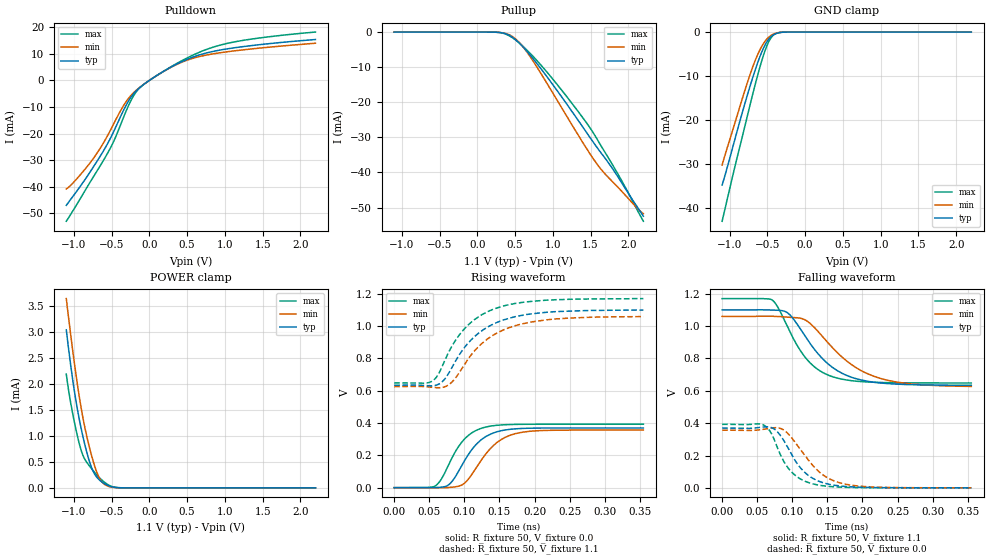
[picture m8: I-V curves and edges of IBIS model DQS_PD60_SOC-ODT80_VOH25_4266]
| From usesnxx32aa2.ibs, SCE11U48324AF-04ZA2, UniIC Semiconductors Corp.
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| DQS_PD60_SOC-ODT80_VOH25_4266
| (60 Ohm Pulldown, 80 Ohm System ODT Setting, VOH=VDDQ/2.5, 3200-4266Mbps)
[Model]   DQS_PD60_SOC-ODT80_VOH25_4266
Model_type   I/O
Vinl = 160.000mV
Vinh = 280.000mV
Vmeas = 220.000mV
Vref = 0.0mV
Cref = 0.0pF
Rref = 80.000Ohm
|   typ   min   max
|C_comp   0.838pF   0.788pF   0.888pF
C_comp_pullup   0.4190pF   0.3940pF   0.4440pF
C_comp_pulldown   0.4190pF   0.3940pF   0.4440pF
| Note: C_comp changes when the ODT circuit is enabled.
[Model Spec]
| Input threshold voltage corners
Vinl   0.1600V   0.1520V   0.1740V
Vinh   0.2800V   0.2720V   0.2940V
| Measurement voltage corners
Vmeas   0.2200V   0.2120V   0.2340V
| Timing spec test load voltage corners
Vref   0.0000V   0.0000V   0.0000V
| Dynamic Overshoot Parameters from LPDDR4 Specification
D_overshoot_ampl_h   0.30   NA   NA
D_overshoot_ampl_l   0.30   NA   NA
D_overshoot_area_h   0.1n   NA   NA
D_overshoot_area_l   0.1n   NA   NA
[Receiver Thresholds]
Vcross_low   = 160.0mV
Vcross_high  = 280.0mV
Vdiff_ac   = 120mV
Vdiff_dc   = 120mV
Tdiffslew_ac = 10.000ns |Not specified, so set to high value
[Voltage Range]   1.1000V   1.0600V   1.1700V
[Pullup Reference]   1.1000V   1.0600V   1.1700V
| Junction Temperature (Ambient temp is 35C typ 95C min -40C max)
[Temperature Range]   50.0   110.0   -40.0
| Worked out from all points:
|   slope of the pulldown table from 0 to 0.165 V, typ, clamps not added: 54.7 ohm
|   slope of the pullup table from 0 to 0.165 V, typ, clamps not added: 16.4 kohm
|   GND clamp passes 1 mA (typ) near -0.45 V on its own axis
|   POWER clamp passes 1 mA (typ) near -0.88 V on its own axis
|   rising waveform, R_fixture 50, V_fixture 0.0: 20-80 % time 35.8ps typ, 39.3ps min, 32.8ps max; typ from 0.001 V to 0.37 V
|   falling waveform, R_fixture 50, V_fixture 1.1: 20-80 % time 55.5ps typ, 67.8ps min, 44.8ps max; typ from 1.1 V to 0.634 V
|   rising waveform, R_fixture 50, V_fixture 1.1: 20-80 % time 57.8ps typ, 60.8ps min, 54.6ps max; typ from 0.634 V to 1.1 V
|   falling waveform, R_fixture 50, V_fixture 0.0: 20-80 % time 36.3ps typ, 43.3ps min, 31.1ps max; typ from 0.37 V to 0.001 V
[Pulldown]
|   Voltage   I(typ)   I(min)   I(max)
-1.1V     -46.99mA   -40.8mA    -52.96mA
-786.5mV  -34.49mA   -31.05mA   -38.36mA
-641.3mV  -28.08mA   -25.11mA   -31.66mA
-525.8mV  -22.32mA   -19.3mA    -25.97mA
-367.4mV  -12.77mA   -10.72mA   -15.73mA
-258.5mV  -6.989mA   -6.176mA   -8.45mA
-162.8mV  -3.638mA   -3.468mA   -3.924mA
-63.8mV   -1.314mA   -1.293mA   -1.298mA
414.7mV   6.826mA    6.638mA    7.153mA
847mV     10.89mA    9.975mA    12.5mA
1.375V    13.14mA    11.88mA    15.61mA
2.2V      15.36mA    13.96mA    18.16mA
[GND Clamp]
|   Voltage   I(typ)   I(min)   I(max)
-1.1V     -34.89mA   -30.34mA   -43.14mA
-935mV    -24.72mA   -20.96mA   -31.01mA
-803mV    -16.58mA   -13.55mA   -21.77mA
-733.7mV  -12.55mA   -9.876mA   -16.88mA
-667.7mV  -8.943mA   -6.74mA    -12.35mA
-591.8mV  -5.274mA   -3.797mA   -7.53mA
-519.2mV  -2.572mA   -1.835mA   -3.676mA
-463.1mV  -1.239mA   -899.6uA   -1.602mA
-410.3mV  -534.6uA   -395.8uA   -582.2uA
-341mV    -134.1uA   -102.7uA   -114.3uA
-242mV    -10.14uA   -9.274uA   -5.696uA
2.2V      0A         0A         0A
[Pullup]
|   Voltage   I(typ)   I(min)   I(max)
-1.1V     4.112uA    7.441uA    1.363uA
259.6mV   -60.64uA   -60.03uA   -61.53uA
388.3mV   -576.1uA   -480.7uA   -688.2uA
500.5mV   -2.042mA   -1.831mA   -2.144mA
609.4mV   -4.304mA   -4.305mA   -4.133mA
731.5mV   -7.378mA   -7.995mA   -6.76mA
1.045V    -16.3mA    -18.97mA   -14.58mA
1.448V    -28.62mA   -33.18mA   -25.89mA
1.573V    -32.49mA   -37.21mA   -29.99mA
1.695V    -36.01mA   -40.47mA   -34.38mA
1.91V     -42.82mA   -45.28mA   -42.24mA
2.2V      -52.46mA   -51.74mA   -53.91mA
[POWER Clamp]
|   Voltage   I(typ)   I(min)   I(max)
-1.1V     3.036mA    3.636mA    2.186mA
-1.041V   2.347mA    2.931mA    1.626mA
-981.2mV  1.754mA    2.277mA    1.183mA
-911.9mV  1.201mA    1.611mA    764.7uA
-852.5mV  818.9uA    1.149mA    543.6uA
-776.6mV  434.4uA    683.5uA    390.2uA
-710.6mV  232.2uA    359.1uA    273.1uA
-657.8mV  146.8uA    178.8uA    190.7uA
-595.1mV  80.84uA    68.31uA    109.3uA
-492.8mV  18.88uA    11.58uA    24.06uA
-380.6mV  1.613uA    1.137uA    1.355uA
2.2V      0A         0A         0A
[Ramp]
|   typ   min   max
| 20% - 80%
dV/dt_r   221.49m/35.79p   213.85m/39.28p   235.57m/32.78p
dV/dt_f   279.40m/55.49p   259.55m/67.76p   312.92m/44.82p
| 25% - 75%
|dV/dt_r   184.57m/28.53p   178.21m/31.31p   196.31m/26.01p
|dV/dt_f   232.84m/44.18p   216.29m/54.01p   260.77m/35.67p
R_load = 50
[Rising Waveform]
R_fixture = 50
V_fixture = 0.0
|   Time   V(typ)   V(min)   V(max)
0s        730.2uV    596.2uV    535.4uV
57ps      628uV      -32uV      8.022mV
66ps      3.145mV    -449.5uV   46.06mV
76ps      13.79mV    1.109mV    127.9mV
101ps     173.6mV    31.4mV     305.2mV
115ps     259.4mV    110.8mV    350.8mV
130ps     315.2mV    206.2mV    375mV
153ps     353.4mV    299.6mV    388.7mV
183ps     367.1mV    343.9mV    392.6mV
355ps     369.9mV    357mV      393.2mV
[Falling Waveform]
R_fixture   = 50
V_fixture   = 1.1
V_fixture_min = 1.06
V_fixture_max = 1.17
|   Time   V(typ)   V(min)   V(max)
0s        1.1V       1.06V      1.17V
72ps      1.099V     1.061V     1.159V
93ps      1.083V     1.055V     997.2mV
118ps     939.2mV    1.039V     809.2mV
135ps     837.9mV    975.1mV    736.5mV
156ps     748.9mV    872.5mV    689.2mV
192ps     673.9mV    740.1mV    659.2mV
228ps     647.4mV    673.7mV    651.3mV
280ps     637mV      638.6mV    648.9mV
355ps     634.3mV    627.4mV    648.5mV
[Rising Waveform]
R_fixture   = 50
V_fixture   = 1.1
V_fixture_min = 1.06
V_fixture_max = 1.17
|   Time   V(typ)   V(min)   V(max)
0s        634mV      625.3mV    648.4mV
53ps      630.3mV    621.7mV    656.8mV
62ps      637.9mV    618.7mV    696mV
75ps      690.1mV    630mV      815.2mV
87ps      780.8mV    677.2mV    909.7mV
104ps     888.4mV    787.7mV    1.001V
124ps     968.6mV    889.1mV    1.068V
149ps     1.027V     962.8mV    1.116V
222ps     1.087V     1.041V     1.161V
355ps     1.099V     1.059V     1.17V
[Falling Waveform]
R_fixture = 50
V_fixture = 0.0
|   Time   V(typ)   V(min)   V(max)
0s        370mV      357.1mV    393.3mV
56ps      375.5mV    360.3mV    393.7mV
73ps      367.3mV    371.8mV    311.6mV
85ps      312mV      364.5mV    187.2mV
96ps      230.6mV    325.8mV    112.5mV
112ps     122.1mV    234.3mV    54.41mV
130ps     57.18mV    134.8mV    24.25mV
155ps     20.24mV    51.87mV    8.198mV
187ps     5.845mV    15.11mV    2.38mV
355ps     781uV      700uV      555.2uV
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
